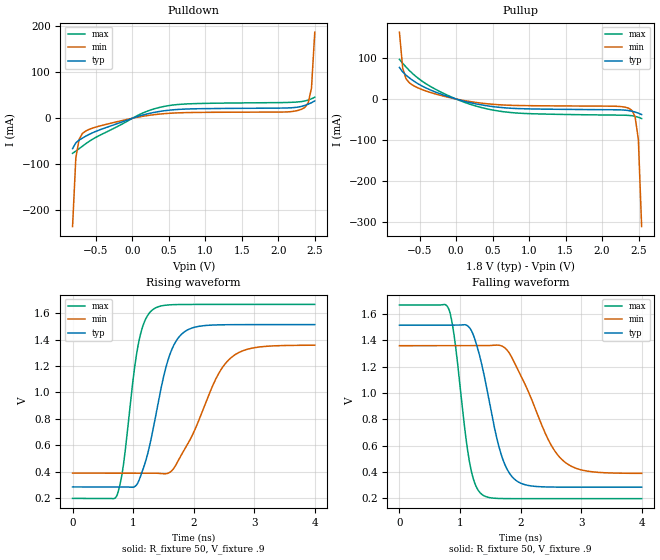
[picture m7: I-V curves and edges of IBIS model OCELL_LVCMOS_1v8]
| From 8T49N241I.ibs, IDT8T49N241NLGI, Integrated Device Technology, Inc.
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[Model] OCELL_LVCMOS_1v8
Model_type   Output
Polarity   Non-Inverting
|   typ   min   max
C_comp   2pF   1.5pF   2.5pF
Vmeas = .9
Rref = 50
Cref = 0
Vref = .9
|   typ   min   max
[Voltage range]   1.8V   1.710V   1.890V
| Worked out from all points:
|   slope of the pulldown table from 0 to 0.27 V, typ, clamps not added: 22.7 ohm
|   slope of the pullup table from 0 to 0.27 V, typ, clamps not added: 23 ohm
|   rising waveform, R_fixture 50, V_fixture .9: 20-80 % time 355ps typ, 571ps min, 238ps max; typ from 0.284 V to 1.51 V
|   falling waveform, R_fixture 50, V_fixture .9: 20-80 % time 350ps typ, 564ps min, 229ps max; typ from 1.51 V to 0.284 V
[Pulldown]
|Voltage   I (typ)   I (min)   I (max)
|Note, modeling breaks down at 250mA and above.  This is well beyond the functional   |
|operating range of the device.  Should this scenario occur, catastrophic failure and   |
|possible damage to the device and/or board is of higher concern than the I-V curve   |
|behavior.  The IBIS checker will flag currents in excess of 10A with warnings.  Lines   |
|with currents in excess of 0.35 A have been commented out.  The points still remain|
|available to the user if the user desires to use them.   |
|-1.64000e+00   -8.47811e+00   -7.79389e+00   -9.69100e+00
|-1.48000e+00   -6.69930e+00   -6.31332e+00   -7.41784e+00
|-1.32000e+00   -4.92075e+00   -4.83297e+00   -5.14538e+00
|-1.16000e+00   -3.14261e+00   -3.35283e+00   -2.87312e+00
|-1.00000e+00   -1.36503e+00   -1.87295e+00   -6.00906e-01
|-9.99000e-01   -1.35392e+00   -1.86370e+00   -5.86705e-01
|-9.54184e-01   -8.56129e-01   -1.44925e+00   -1.60081e-01
|-9.09368e-01   -3.62081e-01   -1.03485e+00   -9.35441e-02
|-8.64552e-01   -1.16470e-01   -6.20514e-01   -8.15268e-02
-819.7mV  -66.02mA   -235.3mA   -76.14mA
-774.9mV  -53.31mA   -86.06mA   -71.33mA
-730.1mV  -47.54mA   -45.74mA   -66.12mA
-685.3mV  -43.08mA   -33.12mA   -60.75mA
-506mV    -28.8mA    -19.43mA   -41.89mA
76.59mV   4.041mA    2.457mA    6.591mA
435.1mV   16.27mA    9.978mA    25.76mA
2.093V    22.29mA    13.65mA    34.21mA
2.317V    25.96mA    19.62mA    36.27mA
2.407V    30.62mA    33.61mA    39.6mA
2.452V    33.81mA    65.56mA    42.31mA
2.497V    37.69mA    186.7mA    45.69mA
| 2.54147e+00   4.28046e-02   6.44034e-01   4.97428e-02
| 2.58629e+00   5.22057e-02   1.45242e+00   5.44736e-02
| 2.63110e+00   8.47753e-02   2.30319e+00   5.97432e-02
| 2.67592e+00   2.46862e-01   3.15402e+00   6.49705e-02
| 2.72074e+00   9.37970e-01   4.00493e+00   6.97810e-02
| 2.76555e+00   1.94925e+00   4.85593e+00   7.69446e-02
| 2.81037e+00   2.97155e+00   5.70702e+00   1.07674e-01
| 2.85518e+00   3.99395e+00   6.55819e+00   3.45229e-01
| 2.90000e+00   5.01646e+00   7.40946e+00   1.42369e+00
| 2.90100e+00   5.03927e+00   7.42846e+00   1.45286e+00
| 3.04080e+00   8.22961e+00   1.00845e+01   5.53179e+00
| 3.18060e+00   1.14210e+01   1.27414e+01   9.61202e+00
| 3.32040e+00   1.46134e+01   1.53991e+01   1.36935e+01
| 3.46020e+00   1.78069e+01   1.80577e+01   1.77762e+01
| 3.60000e+00   2.10014e+01   2.07172e+01   2.18600e+01
[Pullup]
|Voltage   I (typ)   I (min)   I (max)
|Note, modeling breaks down at 250mA and above.  This is well beyond the functional   |
|operating range of the device.  Should this scenario occur, catastrophic failure and   |
|possible damage to the device and/or board is of higher concern than the I-V curve   |
|behavior.  The IBIS checker will flag currents in excess of 10A with warnings.  Lines   |
|with currents in excess of 0.35 A have been commented out.  The points still remain|
|available to the user if the user desires to use them.   |
|-1.64000e+00   1.74090e+01   1.60158e+01   1.98912e+01
|-1.48000e+00   1.37491e+01   1.29694e+01   1.52120e+01
|-1.32000e+00   1.00901e+01   9.92383e+00   1.05337e+01
|-1.16000e+00   6.43209e+00   6.87908e+00   5.85637e+00
|-1.00000e+00   2.77481e+00   3.83505e+00   1.18191e+00
|-9.99000e-01   2.75195e+00   3.81603e+00   1.15371e+00
|-9.54184e-01   1.72764e+00   2.96350e+00   2.80561e-01
|-9.09368e-01   7.38868e-01   2.11098e+00   1.36753e-01
|-8.64552e-01   2.11274e-01   1.25840e+00   1.14150e-01
|-8.19736e-01   1.02225e-01   5.00419e-01   1.04983e-01
-774.9mV  76.7mA     162.1mA    96.32mA
-730.1mV  65.84mA    74.78mA    86.86mA
-685.3mV  58.13mA    49.39mA    77.79mA
-595.7mV  45.73mA    33.89mA    61.96mA
-416.4mV  27.22mA    19.67mA    37.64mA
76.59mV   -3.805mA   -2.678mA   -5.493mA
569.6mV   -19.79mA   -13.68mA   -28.8mA
2.183V    -26.15mA   -17.61mA   -39.08mA
2.407V    -29.63mA   -27.48mA   -40.61mA
2.452V    -31.71mA   -43.12mA   -42.14mA
2.497V    -34.33mA   -98.55mA   -44.44mA
2.541V    -37.73mA   -309.9mA   -47.47mA
| 2.58629e+00   -4.33733e-02   -7.17845e-01   -5.11150e-02
| 2.63110e+00   -5.99455e-02   -1.13158e+00   -5.52160e-02
| 2.67592e+00   -1.34019e-01   -1.54542e+00   -5.94825e-02
| 2.72074e+00   -4.70459e-01   -1.95934e+00   -6.36543e-02
| 2.76555e+00   -9.67588e-01   -2.37333e+00   -6.90194e-02
| 2.81037e+00   -1.46482e+00   -2.78737e+00   -8.55313e-02
| 2.85518e+00   -1.96215e+00   -3.20147e+00   -1.93508e-01
| 2.90000e+00   -2.45958e+00   -3.61562e+00   -7.26898e-01
| 2.90100e+00   -2.47068e+00   -3.62486e+00   -7.41088e-01
| 3.04080e+00   -4.02293e+00   -4.91703e+00   -2.72518e+00
| 3.18060e+00   -5.57585e+00   -6.20957e+00   -4.70971e+00
| 3.32040e+00   -7.12925e+00   -7.50242e+00   -6.69473e+00
| 3.46020e+00   -8.68302e+00   -8.79557e+00   -8.68053e+00
| 3.60000e+00   -1.02371e+01   -1.00890e+01   -1.06670e+01
[Ramp]
|   typ   min   max
dV/dt_r   0.74/0.355n   0.584/0.574n   0.883/0.237n
dV/dt_f   0.74/0.351n   0.584/0.566n   0.885/0.23n
R_load =   50.0000
[Rising Waveform]
R_fixture = 50
V_fixture = .9   |Vcc_typ
V_fixture_min = .855 |Vcc_min
V_fixture_max = .945 |Vcc_max
C_fixture = 0.0p
| Time   typ   min   max
0s        283.8mV    388.4mV    196.6mV
733.3ps   283.9mV    388.4mV    220.2mV
835.6ps   284.1mV    388.4mV    436.6mV
1.084ns   320.3mV    388.5mV    1.362V
1.32ns    698.7mV    388.7mV    1.626V
1.587ns   1.261V     389.6mV    1.664V
1.862ns   1.464V     577.4mV    1.667V
2.378ns   1.512V     1.113V     1.668V
2.636ns   1.514V     1.27V      1.668V
4ns       1.515V     1.358V     1.668V
[Falling Waveform]
R_fixture = 50
V_fixture = .9   |Vcc_typ
V_fixture_min = .855 |Vcc_min
V_fixture_max = .945 |Vcc_max
C_fixture = 0.0p
| Time   typ   min   max
0s        1.515V     1.359V     1.668V
813.3ps   1.515V     1.359V     1.639V
911.1ps   1.514V     1.359V     1.411V
1.156ns   1.496V     1.359V     479.8mV
1.36ns    1.216V     1.358V     229.8mV
1.667ns   553.4mV    1.36V      197.7mV
1.924ns   335.7mV    1.206V     196.7mV
2.458ns   285.3mV    645.2mV    196.6mV
2.711ns   284.1mV    482.3mV    196.6mV
4ns       283.8mV    388.8mV    196.6mV
